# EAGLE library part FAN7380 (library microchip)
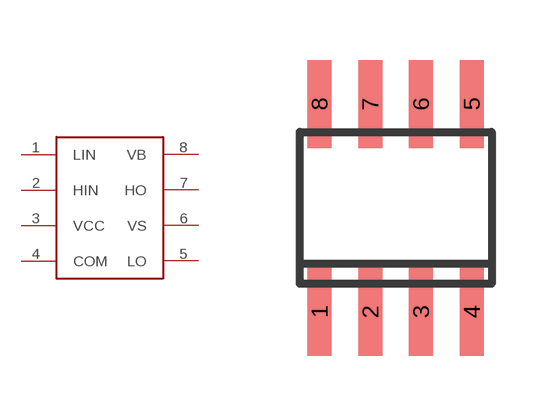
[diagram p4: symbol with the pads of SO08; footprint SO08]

Designator prefix -

## FAN7380  [SO08]
1  LIN
2  HIN
3  VCC
4  COM
5  LO
6  VS
7  HO
8  VB

## Footprint SO08 (pad centres in mm)
Small Outline Package
smd 0.6 x 2.2: 1 -1.905,-2.6; 2 -0.635,-2.6; 3 0.635,-2.6; 4 1.905,-2.6; 5 1.905,2.6; 6 0.635,2.6; 7 -0.635,2.6; 8 -1.905,2.6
